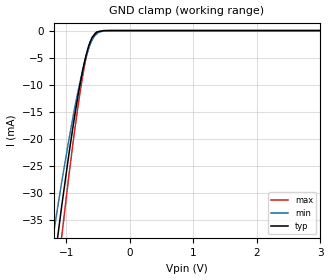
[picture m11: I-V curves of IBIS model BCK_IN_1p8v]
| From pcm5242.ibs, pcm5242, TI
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|   BCK_IN_1p8v
[Model]   BCK_IN_1p8v
Model_type   Input
Vinl = 0.54
Vinh = 1.26
|   typ   min   max
C_comp   1.514291423pF   1.436730626pF   1.542051917pF
[Voltage Range]   1.8   1.65   1.95
[Temperature Range]   27   105   -25
[Power Clamp Reference]   1.8   1.65   1.95
[GND Clamp Reference]   -0   -0   -0
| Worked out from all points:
|   GND clamp passes 1 mA (typ) near -0.57 V on its own axis
[GND Clamp]
|   Voltage   I(typ)   I(min)   I(max)
-1.8V     -103.9mA   -86.97mA   -120.1mA
-1.29V    -52.65mA   -44.58mA   -61.57mA
-1.182V   -42.49mA   -36.24mA   -49.8mA
-1.074V   -32.76mA   -28.25mA   -38.44mA
-974.7mV  -24.27mA   -21.3mA    -28.44mA
-880.4mV  -16.79mA   -15.16mA   -19.63mA
-734.2mV  -6.985mA   -6.98mA    -7.926mA
-686.2mV  -4.486mA   -4.819mA   -4.945mA
-622.6mV  -2.125mA   -2.565mA   -2.05mA
-539.6mV  -557.4uA   -827.2uA   -348.4uA
-296.6mV  -421.6nA   -3.207uA   -166.4nA
3.6V      0A         0A         0A
[POWER Clamp]
|   Voltage   I(typ)   I(min)   I(max)
-1.8V     0A         0A         0A
0V        0A         0A         0A
3.6V      0A         0A         0A
